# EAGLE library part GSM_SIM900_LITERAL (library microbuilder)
SIM900 Quad-Band GSM/GPRS Module Power Supply: 3.2-4.8V Temperature Range: -30°C-+80°C Bands: GSM 850, EGSM 900, DCS 1800, PCS 1900
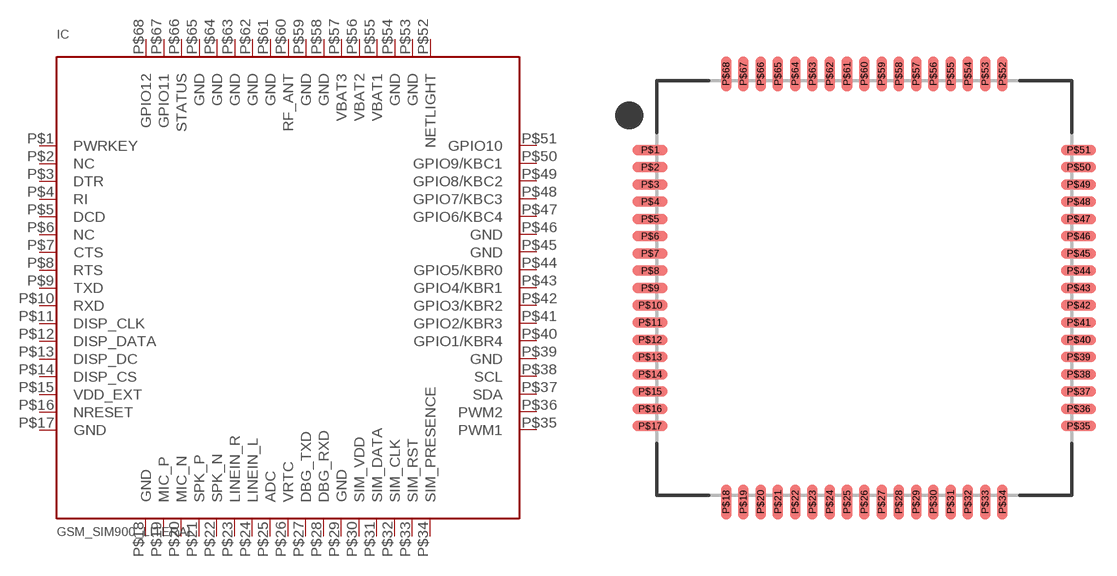
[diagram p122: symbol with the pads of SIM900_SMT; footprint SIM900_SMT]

Designator prefix IC

## GSM_SIM900_LITERAL  [SIM900_SMT]
P$1  PWRKEY  pwr
P$2  NC  nc
P$3  DTR  in
P$4  RI  out
P$5  DCD  out
P$6  NC  nc
P$7  CTS  out
P$8  RTS  in
P$9  TXD  out
P$10  RXD  in
P$11  DISP_CLK
P$12  DISP_DATA
P$13  DISP_DC
P$14  DISP_CS
P$15  VDD_EXT
P$16  NRESET
P$17  GND  pwr
P$18  GND  pwr
P$19  MIC_P
P$20  MIC_N
P$21  SPK_P
P$22  SPK_N
P$23  LINEIN_R
P$24  LINEIN_L
P$25  ADC
P$26  VRTC  pwr
P$27  DBG_TXD  out
P$28  DBG_RXD  in
P$29  GND  pwr
P$30  SIM_VDD  pwr
P$31  SIM_DATA
P$32  SIM_CLK
P$33  SIM_RST
P$34  SIM_PRESENCE
P$35  PWM1
P$36  PWM2
P$37  SDA
P$38  SCL
P$39  GND  pwr
P$40  GPIO1/KBR4
P$41  GPIO2/KBR3
P$42  GPIO3/KBR2
P$43  GPIO4/KBR1
P$44  GPIO5/KBR0
P$45  GND  pwr
P$46  GND  pwr
P$47  GPIO6/KBC4
P$48  GPIO7/KBC3
P$49  GPIO8/KBC2
P$50  GPIO9/KBC1
P$51  GPIO10
P$52  NETLIGHT
P$53  GND  pwr
P$54  GND  pwr
P$55  VBAT1  pwr
P$56  VBAT2  pwr
P$57  VBAT3  pwr
P$58  GND  pwr
P$59  GND  pwr
P$60  RF_ANT
P$61  GND  pwr
P$62  GND  pwr
P$63  GND  pwr
P$64  GND  pwr
P$65  GND  pwr
P$66  STATUS
P$67  GPIO11  pwr
P$68  GPIO12  pwr

## Footprint SIM900_SMT (pad centres in mm)
smd 2 x 0.6: P$1 -12.4,8; P$2 -12.4,7; P$3 -12.4,6; P$4 -12.4,5; P$5 -12.4,4; P$6 -12.4,3; P$7 -12.4,2; P$8 -12.4,1; P$9 -12.4,0; P$10 -12.4,-1; P$11 -12.4,-2; P$12 -12.4,-3; P$13 -12.4,-4; P$14 -12.4,-5; P$15 -12.4,-6; P$16 -12.4,-7; P$17 -12.4,-8; P$35 12.4,-8; P$36 12.4,-7; P$37 12.4,-6; P$38 12.4,-5; P$39 12.4,-4; P$40 12.4,-3; P$41 12.4,-2; P$42 12.4,-1; P$43 12.4,0; P$44 12.4,1; P$45 12.4,2; P$46 12.4,3; P$47 12.4,4; P$48 12.4,5; P$49 12.4,6; P$50 12.4,7; P$51 12.4,8
smd 0.6 x 2: P$18 -8,-12.4; P$19 -7,-12.4; P$20 -6,-12.4; P$21 -5,-12.4; P$22 -4,-12.4; P$23 -3,-12.4; P$24 -2,-12.4; P$25 -1,-12.4; P$26 0,-12.4; P$27 1,-12.4; P$28 2,-12.4; P$29 3,-12.4; P$30 4,-12.4; P$31 5,-12.4; P$32 6,-12.4; P$33 7,-12.4; P$34 8,-12.4; P$52 8,12.4; P$53 7,12.4; P$54 6,12.4; P$55 5,12.4; P$56 4,12.4; P$57 3,12.4; P$58 2,12.4; P$59 1,12.4; P$60 0,12.4; P$61 -1,12.4; P$62 -2,12.4; P$63 -3,12.4; P$64 -4,12.4; P$65 -5,12.4; P$66 -6,12.4; P$67 -7,12.4; P$68 -8,12.4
